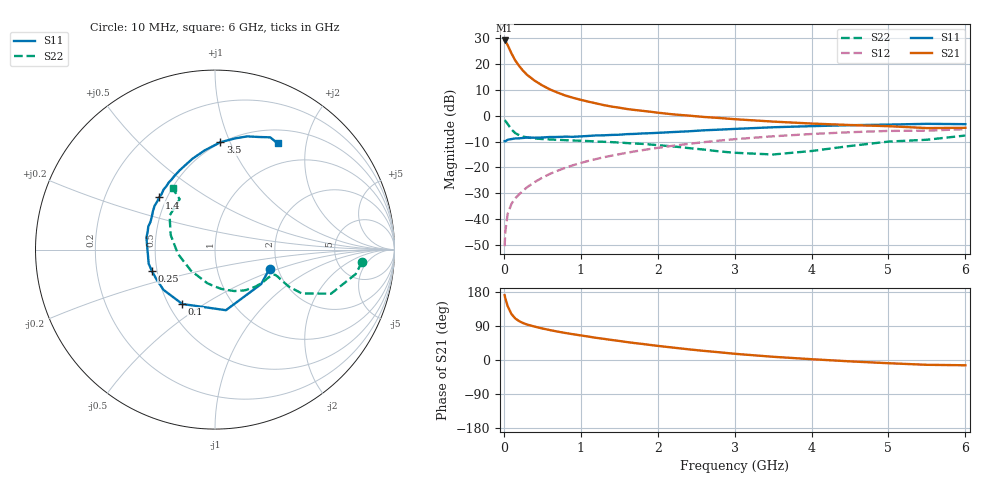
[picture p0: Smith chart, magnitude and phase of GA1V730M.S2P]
! Infineon Technologies  Discrete & RF Semiconductors
! BF775
! Si NPN RF Bipolar Junction Transistor in SOT23
! VCE = 1.75 V  IC = 30 mA
! Common Emitter S-Parameters:  May  1996
# GHz  S  MA  R  50
!  f  S11  S21  S12  S22
! GHz  MAG  ANG  MAG  ANG  MAG  ANG  MAG  ANG
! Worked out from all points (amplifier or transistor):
!   36 points, 10 MHz to 6 GHz, reference 50 ohm
!   highest |S21| = 29.1 dB at 10 MHz (marker M1)
!   |S21| within 3 dB of that: start of sweep to 68.26 MHz
!   unconditionally stable (mu >= 1): start of sweep to 20.95 MHz; 109.1 MHz to end of sweep
!   at 250 MHz: K = 1.37, MAG = 19.6 dB, |S12| = -29.0 dB
!   at 1.4 GHz: K = 1.46, MAG = 5.5 dB, |S12| = -15.5 dB
!   at 6 GHz: K = 1.11, MAG = -1.8 dB, |S12| = -5.2 dB
!   S11 on the Smith chart (normalised r, x): 10 MHz: 1.81, -0.43; 100 MHz: 0.59, -0.41; 250 MHz: 0.47, -0.13; 1.4 GHz: 0.45, +0.32; 3.5 GHz: 0.49, +0.92; 6 GHz: 0.68, +1.53
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0.01  0.3223 -19.4  28.56 171.0  0.003 79.9  0.8228 -4.8
0.02  0.321 -36.8  27.63 162.4  0.0059 79.2  0.795 -9.9
0.05  0.3431 -79.8  23.14 141.7  0.0127 67.1  0.6917 -20.8
0.1  0.3536 -121.0  15.99 121.0  0.0199 61.8  0.5415 -26.8
0.15  0.3643 -142.0  11.62 109.3  0.0254 62.3  0.4593 -26.6
0.2  0.3657 -153.1  9.138 102.4  0.0303 64.9  0.42 -25.2
0.25  0.3716 -161.6  7.405 97.5  0.0354 66.7  0.3956 -24.1
0.3  0.3777 -168.0  6.214 93.7  0.0412 68.5  0.3811 -23.3
0.4  0.3752 -177.4  4.772 88.2  0.052 70.4  0.3637 -22.8
0.5  0.3797 176.0  3.854 83.2  0.0633 71.3  0.354 -23.2
0.6  0.3878 170.0  3.225 78.9  0.0751 71.2  0.3476 -24.3
0.7  0.3885 164.8  2.793 74.9  0.0865 71.5  0.3424 -25.8
0.8  0.3933 160.9  2.458 71.3  0.0983 70.7  0.3366 -27.5
1.1  0.4066 148.3  1.87 61.8  0.134 68.5  0.3233 -33.8
1.4  0.4253 136.9  1.505 52.9  0.1687 65.3  0.3086 -40.8
1.7  0.4451 127.5  1.293 44.7  0.204 61.9  0.2898 -48.7
2.2  0.4834 114.1  1.063 32.7  0.2627 55.3  0.2551 -64.9
3  0.5559 95.9  0.857 16.4  0.3517 43.5  0.1922 -102.9
3.5  0.5985 87.2  0.77 8.5  0.4003 35.8  0.1779 -138.8
4.5  0.6559 74.1  0.661 -3.6  0.4798 20.5  0.2598 161.8
5.5  0.6971 63.8  0.577 -12.7  0.5139 5.3  0.3434 125.0
6  0.6868 59.4  0.584 -13.9  0.5504 1.1  0.4141 124.7
